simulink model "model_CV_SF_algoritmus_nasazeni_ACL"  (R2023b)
settings: Solver=FixedStepAuto  StartTime=0.0  StopTime=inf  RelTol=1e-3  EnableMultiTasking=on
libraries: visiontextngfix x3, raspberrypiAVlib x2, lib_control_system_SF x1, deeplib x1, dspstat3 x1, raspberrypiBasiclib x1

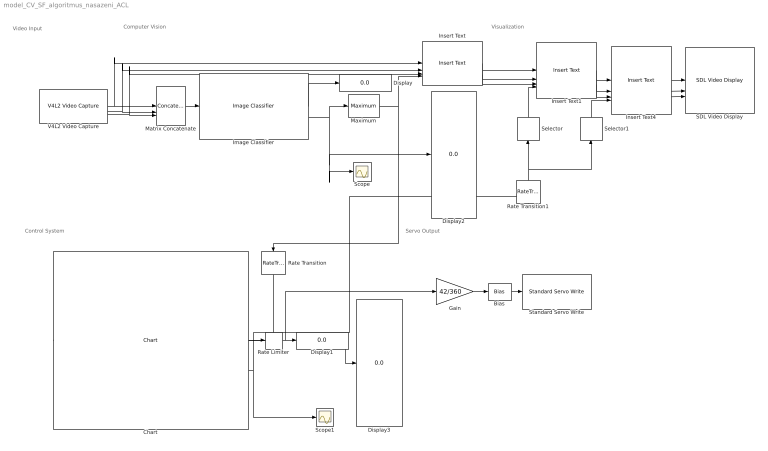
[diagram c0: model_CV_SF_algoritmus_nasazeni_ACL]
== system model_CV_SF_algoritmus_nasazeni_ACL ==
  note: Video Input
  note: Servo Output
  note: Control System
  note: Computer Vision
  note: Visualization
  Bias : Bias  Bias=2
  Chart : lib_control_system_SF/Chart  SystemSampleTime=-1  VariantActivationTime=update diagram  AllowFlexibleInterface=on  Latency=0  AutoFrameSizeCalculation=off
  Display{,1..3} (4 alike) : Display
  Gain : Gain  Gain=42/360
  Image Classifier : deeplib/Image Classifier  Network=Network from MAT-file  NetworkFunction=squeezenet  NetworkFilePath=trainedNetwork.mat  MiniBatchSize=8  ResizeInput=on  Classification=on  Predictions=on  ForceInterpretedSim=off  PredictMode=All probabilities and labels  K=5
  Insert Text : visiontextngfix/Insert Text  inputType=Obsolete  theText={'Hmozdinka','Hrebik','Matice','Matice kridlova','Podlozka','Prazdne','Sroub','Vrut'}  getTextLocFrom=Specify via dialog  textLoc=[1 1]  getTextColorFrom=Specify via dialog  textColor=[0 0 0]  getTextIntensityFrom=Specify via dialog  textIntensity=0  getTextOpacityFrom=Specify via dialog  textOpacity=1.0  dummyVar2=0  dummyVar3=0  dummyVar4=0  imagePorts=Separate color signals  isInputTransposed=on  fontFace=LucidaSansRegular  dummyVar1=0  blockFontSize=32  antiAliased=on
  Insert Text1 : visiontextngfix/Insert Text  inputType=Obsolete  theText='Hm: %3.0f, Hr: %3.0f, Ma: %3.0f, MaK: %3.0f'  getTextLocFrom=Specify via dialog  textLoc=[1 200]  getTextColorFrom=Specify via dialog  textColor=[0 0 0]  getTextIntensityFrom=Specify via dialog  textIntensity=0  getTextOpacityFrom=Specify via dialog  textOpacity=1.0  dummyVar2=0  dummyVar3=0  dummyVar4=0  imagePorts=Separate color signals  isInputTransposed=on  fontFace=LucidaSansRegular  dummyVar1=0  blockFontSize=18  antiAliased=on
  Insert Text4 : visiontextngfix/Insert Text  inputType=Obsolete  theText='Po: %3.0f, Sr: %3.0f, Vr: %3.0f'  getTextLocFrom=Specify via dialog  textLoc=[1 220]  getTextColorFrom=Specify via dialog  textColor=[0 0 0]  getTextIntensityFrom=Specify via dialog  textIntensity=0  getTextOpacityFrom=Specify via dialog  textOpacity=1.0  dummyVar2=0  dummyVar3=0  dummyVar4=0  imagePorts=Separate color signals  isInputTransposed=on  fontFace=LucidaSansRegular  dummyVar1=0  blockFontSize=18  antiAliased=on
  Matrix Concatenate : Concatenate  NumInputs=3  Mode=Multidimensional array  ConcatenateDimension=3
  Maximum : dspstat3/Maximum  operation=maximum  fcn=Index  indexBase=One  operateOver=Each row  Dimension=1  InputProcessing=Columns as channels (frame based)  reset=None  roiEnable=off  roiType=Rectangles  roiPortion=Entire ROI  roiOutput=Individual statistics for each ROI  roiFlag=off  roundingMode=Floor  overflowMode=off  accumDataTypeStr=Inherit: Same as product output  accumLastDataTypeStr=Inherit: Same as product output
  Rate Limiter : RateLimiter  RisingSlewLimit=15  FallingSlewLimit=-15  SampleTimeMode=inherited
  Rate Transition : RateTransition  OutPortSampleTime=0.1
  Rate Transition1 : RateTransition  OutPortSampleTime=0.2
  SDL Video Display : raspberrypiAVlib/SDL Video Display  title=SDL Video Display  pixelFormat=RGB  pixelOrder=Planar  rowMajor=on  blockPlatform=Raspberry Pi
  Scope : Scope
  Scope1 : Scope
  Selector : Selector  InputPortWidth=8  IndexOptions=Index vector (dialog)  Indices=1:4  OutputSizes=1
  Selector1 : Selector  InputPortWidth=8  IndexOptions=Index vector (dialog)  Indices=[5 7 8]  OutputSizes=1
  Standard Servo Write : raspberrypiBasiclib/Standard Servo Write  board=Pi 2 Model B  Pin_=18  MinPulseDuration=1000e-6  MaxPulseDuration=2000e-6  blockPlatform=Raspberry Pi
  V4L2 Video Capture : raspberrypiAVlib/V4L2 Video Capture  DeviceName=/dev/video0  Resolution=320x240  CustomResolution=[ 320, 240 ]  PixelFormat=RGB  SampleTime=0.2  pixelOrder=planar  simOutput=Colorbars  imSizeSelection=320x240  imSize=[640, 480]  roi=[0, 0, 640, 480]  m_devName='/dev/video0'  blockPlatform=LINUX  HorizontalFlip=off  VerticalFlip=off  Brightness=0.0  Saturation=0.25  Contrast=0.5  Sharpness=0.5  CameraPan=0  CameraTilt=0  CameraZoom=0.5  EnableManualFocus=on  ManualFocus=0.5
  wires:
  Image Classifier/1 -> Display/1
  Image Classifier/2 -> Maximum/1, Scope/1, Display2/1
  Insert Text/1 -> Insert Text1/1
  Maximum/1 -> Insert Text/4, Rate Transition/1
  Chart/1 -> Rate Limiter/1
  Chart/2 -> Rate Transition1/1, Display3/1, Scope1/1
  Gain/1 -> Bias/1
  Bias/1 -> Standard Servo Write/1
  Insert Text/2 -> Insert Text1/2
  Insert Text/3 -> Insert Text1/3
  V4L2 Video Capture/1 -> Insert Text/1, Matrix Concatenate/1
  V4L2 Video Capture/2 -> Matrix Concatenate/2, Insert Text/2
  V4L2 Video Capture/3 -> Matrix Concatenate/3, Insert Text/3
  Matrix Concatenate/1 -> Image Classifier/1
  Rate Limiter/1 -> Gain/1, Display1/1
  Insert Text1/1 -> Insert Text4/1
  Insert Text4/1 -> SDL Video Display/1
  Insert Text4/2 -> SDL Video Display/2
  Insert Text4/3 -> SDL Video Display/3
  Selector/1 -> Insert Text1/4
  Selector1/1 -> Insert Text4/4
  Insert Text1/2 -> Insert Text4/2
  Insert Text1/3 -> Insert Text4/3
  Rate Transition/1 -> Chart/1
  Rate Transition1/1 -> Selector/1, Selector1/1
